| z11b.ibs * IBIS 7.0 Model
| 8Gb DDR4 SDRAM - Die Revision "E"
| This Model is valid for Commercial Temperature Range 0C<=Tc<=95C
| Valid for DDR4-1600/1866/2133/2400/2666/2933/3200 operation
| Models *_3200 are applicable for speed grade 3200 Mbps (-062) and below
| Part Number   VDD/VDDQ   Architecture   Package
| MT40A2G4SA   1.2V/1.2V   2Gb   x 4   78-Ball FBGA
| MT40A1G8SA   1.2V/1.2V   1Gb   x 8   78-Ball FBGA
| MT40A512M16LY   1.2V/1.2V   512Mb x 16   96-Ball FBGA
| MT40A2G4Z11B   1.2V/1.2V   2Gb   x 4   Bare Die
| MT40A1G8Z11B   1.2V/1.2V   1Gb   x 8   Bare Die
| MT40A512M16Z11B   1.2V/1.2V   512Mb x 16   Bare Die
[IBIS Ver]   7.0
[File Name]   z11b.ibs
[Date]   2/27/2023
[File Rev]   2.9.2
[Source]   From silicon level SPICE model at Micron Technology, Inc.
   For support contact your local Micron FAE/Sales contacts
   (more information at https://www.micron.com/support/sales-network)
[Notes]   Revision History:
   Rev 2.9.2: 2/27/2023
   - Updated bare die components and pin mapping tables
   Notes:
   - The DQ_IN_ODT* models contain assumed input thresholds,
   the actual threshold values will depend on the VREFDQ
   level set by training
   - This IBIS file uses the Submodel keyword to model the
   DDR4 On-die Termination(ODT) characteristics.
   - The C_comp value in the DQ I/O model is set to match the
   input state of the DQ I/O as measured from the HSPICE model.
   The C_comp value decreases in the DQ/DQS Input ODT models.
   - L_pin values in the Pin sections are loop inductance and
   include the mutual inductance to appropriate POWER/GND
   return paths.  POWER/GND parasitics are modeled in the
   Package Models.
   - Typ and slow corner V-t curves in the following DQ* models
   are shifted relative to strong corner V-t curve
   to contain all 3 corners within appropriate V-t window
   Models   Typ   Slow   V-t duration
   DQ*_34_3200   -100ps   -250ps   500ps
   DQ*_40_3200   -100ps   -250ps   500ps
   DQ*_48_3200   -100ps   -250ps   500ps
   ALERT_3200   -70ps   -180ps   500ps
   - Due to the shift in typ and slow corner, the V-t curves
   may overlap each other. This does not effect the accuracy
   of the IBIS data.
   - The NF_INPUT Model is for Non-functioning pins in the x4
   package
   - The NF_DQ Model is for Non-functioning DQ pins in the
   x4 package
   See Micron IBIS Model Quality Report and Quality Checklist
   for full IQ details
[Disclaimer]  This software code and all associated documentation, comments
   or other information (collectively "Software") is provided
   "AS IS" without warranty of any kind. MICRON TECHNOLOGY, INC.
   ("MTI") EXPRESSLY DISCLAIMS ALL WARRANTIES EXPRESS OR IMPLIED,
   INCLUDING BUT NOT LIMITED TO, NONINFRINGEMENT OF THIRD PARTY
   RIGHTS, AND ANY IMPLIED WARRANTIES OF MERCHANTABILITY OR
   FITNESS FOR ANY PARTICULAR PURPOSE. MTI DOES NOT WARRANT THAT
   THE SOFTWARE WILL MEET YOUR REQUIREMENTS, OR THAT THE
   OPERATION OF THE SOFTWARE WILL BE UNINTERRUPTED OR ERROR-FREE.
   FURTHERMORE, MTI DOES NOT MAKE ANY REPRESENTATIONS REGARDING
   THE USE OR THE RESULTS OF THE USE OF THE SOFTWARE IN TERMS OF
   ITS CORRECTNESS, ACCURACY, RELIABILITY, OR OTHERWISE. THE
   ENTIRE RISK ARISING OUT OF USE OR PERFORMANCE OF THE SOFTWARE
   REMAINS WITH YOU. IN NO EVENT SHALL MTI, ITS AFFILIATED
   COMPANIES OR THEIR SUPPLIERS BE LIABLE FOR ANY DIRECT,
   INDIRECT, CONSEQUENTIAL, INCIDENTAL, OR SPECIAL DAMAGES
   (INCLUDING, WITHOUT LIMITATION, DAMAGES FOR LOSS OF PROFITS,
   BUSINESS INTERRUPTION, OR LOSS OF INFORMATION) ARISING OUT OF
   YOUR USE OF OR INABILITY TO USE THE SOFTWARE, EVEN IF MTI HAS
   BEEN ADVISED OF THE POSSIBILITY OF SUCH DAMAGES. Because some
   jurisdictions prohibit the exclusion or limitation of
   liability for consequential or incidental damages, the above
   limitation may not apply to you.
[Copyright]   Copyright 2023 Micron Technology, Inc. All rights reserved.
| COMPONENT: MT40A2G4SA (78-Ball FBGA, x4)
[Component]   MT40A2G4SA
[Package Model] z11b_78ball_pkg
[Manufacturer]  Micron Technology,Inc.
[Package]
|   typ   min   max
R_pkg   0.420   0.337   0.508
L_pkg   1.872nH   1.600nH   2.256nH
C_pkg   0.503pF   0.373pF   0.869pF
[Pin]   signal_name   model_name   R_pin   L_pin   C_pin   | TD_pin(ps)   Z_pin
A1   VDD   POWER
A2   VSS   GND
A3   NF   NF_DQ   0.468   1.674nH   0.508pF   | 29.160   57.411
A7   NF   NF_DQ   0.479   1.742nH   0.585pF   | 31.921   54.584
A8   VSS   GND
A9   VSS   GND
B1   VPP   POWER
B2   VDDQ   POWER
B3   DQS_c   DQS   0.483   1.679nH   0.529pF   | 29.803   56.344
B7   DQ1   DQ   0.467   1.632nH   0.584pF   | 30.879   52.837
B8   VDDQ   POWER
B9   ZQ   NC
C1   VDDQ   POWER
C2   DQ0   DQ   0.469   1.610nH   0.574pF   | 30.404   52.960
C3   DQS_t   DQS   0.475   1.798nH   0.476pF   | 29.260   61.450
C7   VDD   POWER
C8   VSS   GND
C9   VDDQ   POWER
D1   VSS   GND
D2   NC   NC
D3   DQ2   DQ   0.471   1.737nH   0.510pF   | 29.758   58.380
D7   DQ3   DQ   0.464   1.678nH   0.578pF   | 31.131   53.899
D8   NC   NC
D9   VSS   GND
E1   VSSL   GND
E2   VDDQ   POWER
E3   NC   NC
E7   NC   NC
E8   VDDQ   POWER
E9   VSS   GND
F1   VDDL   POWER
F2   NC   NC
F3   ODT   INPUT   0.423   2.049nH   0.469pF   | 30.987   66.123
F7   CK_t   CLKIN   0.424   1.731nH   0.474pF   | 28.640   60.452
F8   CK_c   CLKIN   0.419   1.671nH   0.528pF   | 29.696   56.277
F9   VDD   POWER
G1   VSS   GND
G2   NC   NC
G3   CKE   INPUT   0.417   2.095nH   0.424pF   | 29.791   70.324
G7   CS_n   INPUT   0.417   1.902nH   0.442pF   | 29.003   65.579
G8   NC   NC
G9   TEN   INPUT   0.402   2.078nH   0.888pF   | 42.963   48.376
H1   VDD   POWER
H2   WE_n_A14   INPUT   0.406   2.014nH   0.473pF   | 30.864   65.258
H3   ACT_n   INPUT   0.408   1.881nH   0.419pF   | 28.078   66.976
H7   CAS_n_A15   INPUT   0.405   1.965nH   0.393pF   | 27.777   70.734
H8   RAS_n_A16   INPUT   0.412   1.989nH   0.479pF   | 30.861   64.442
H9   VSS   GND
J1   VREFCA   POWER
J2   BG0   INPUT   0.406   1.898nH   0.453pF   | 29.337   64.694
J3   A10   INPUT   0.406   1.830nH   0.393pF   | 26.827   68.213
J7   A12_BC_n   INPUT   0.406   1.941nH   0.378pF   | 27.084   71.672
J8   BG1   INPUT   0.418   2.042nH   0.470pF   | 30.983   65.919
J9   VDD   POWER
K1   VSS   GND
K2   BA0   INPUT   0.409   1.979nH   0.487pF   | 31.052   63.720
K3   A4   INPUT   0.407   1.854nH   0.438pF   | 28.491   65.085
K7   A3   INPUT   0.405   1.944nH   0.427pF   | 28.818   67.441
K8   BA1   INPUT   0.406   2.024nH   0.474pF   | 30.975   65.344
K9   VSS   GND
L1   RESET_n   INPUT   0.352   1.673nH   0.740pF   | 35.197   47.547
L2   A6   INPUT   0.405   1.847nH   0.490pF   | 30.073   61.424
L3   A0   INPUT   0.405   1.689nH   0.426pF   | 26.827   62.951
L7   A1   INPUT   0.409   1.872nH   0.430pF   | 28.361   66.019
L8   A5   INPUT   0.410   1.932nH   0.502pF   | 31.135   62.058
L9   ALERT_n   ALERT   0.348   1.777nH   0.723pF   | 35.847   49.561
M1   VDD   POWER
M2   A8   INPUT   0.409   1.918nH   0.485pF   | 30.505   62.883
M3   A2   INPUT   0.414   1.875nH   0.410pF   | 27.733   67.600
M7   A9   INPUT   0.411   1.946nH   0.399pF   | 27.864   69.857
M8   A7   INPUT   0.410   1.997nH   0.497pF   | 31.507   63.393
M9   VPP   POWER
N1   VSS   GND
N2   A11   INPUT   0.405   1.872nH   0.506pF   | 30.765   60.840
N3   PARITY   INPUT   0.411   1.710nH   0.481pF   | 28.673   59.651
N7   NC   NC
N8   A13   INPUT   0.416   2.062nH   0.486pF   | 31.647   65.172
N9   VDD   POWER
|***********************PIN MAPPING*****************************************
[Pin Mapping]   pulldown_ref   pullup_ref   gnd_clamp_ref   power_clamp_ref ext_ref
A1   NC   VDD
A2   VSS   NC
A3   NC   NC   VSS   VDDQ
A7   NC   NC   VSS   VDDQ
A8   VSS   NC
A9   VSS   NC
B1   NC   VPP
B2   NC   VDDQ
B3   VSS   VDDQ   VSS   VDDQ
B7   VSS   VDDQ   VSS   VDDQ
B8   NC   VDDQ
B9   NC   NC
C1   NC   VDDQ
C2   VSS   VDDQ   VSS   VDDQ
C3   VSS   VDDQ   VSS   VDDQ
C7   NC   VDD
C8   VSS   NC
C9   NC   VDDQ
D1   VSS   NC
D2   NC   NC
D3   VSS   VDDQ   VSS   VDDQ
D7   VSS   VDDQ   VSS   VDDQ
D8   NC   NC
D9   VSS   NC
E1   VSSL   NC
E2   NC   VDDQ
E3   NC   NC
E7   NC   NC
E8   NC   VDDQ
E9   VSS   NC
F1   NC   VDDL
F2   NC   NC
F3   NC   NC   VSS   VDD
F7   NC   NC   VSS   VDD
F8   NC   NC   VSS   VDD
F9   NC   VDD
G1   VSS   NC
G2   NC   NC
G3   NC   NC   VSS   VDD
G7   NC   NC   VSS   VDD
G8   NC   NC
G9   NC   NC   VSS   VDD
H1   NC   VDD
H2   NC   NC   VSS   VDD
H3   NC   NC   VSS   VDD
H7   NC   NC   VSS   VDD
H8   NC   NC   VSS   VDD
H9   VSS   NC
J1   NC   VREFCA
J2   NC   NC   VSS   VDD
J3   NC   NC   VSS   VDD
J7   NC   NC   VSS   VDD
J8   NC   NC   VSS   VDD
J9   NC   VDD
K1   VSS   NC
K2   NC   NC   VSS   VDD
K3   NC   NC   VSS   VDD
K7   NC   NC   VSS   VDD
K8   NC   NC   VSS   VDD
K9   VSS   NC
L1   NC   NC   VSS   VDD
L2   NC   NC   VSS   VDD
L3   NC   NC   VSS   VDD
L7   NC   NC   VSS   VDD
L8   NC   NC   VSS   VDD
L9   VSS   VDDQ   VSS   VDDQ
M1   NC   VDD
M2   NC   NC   VSS   VDD
M3   NC   NC   VSS   VDD
M7   NC   NC   VSS   VDD
M8   NC   NC   VSS   VDD
M9   NC   VPP
N1   VSS   NC
N2   NC   NC   VSS   VDD
N3   NC   NC   VSS   VDD
N7   NC   NC
N8   NC   NC   VSS   VDD
N9   NC   VDD
|**********************DIFF PIN*********************************************
[Diff_pin]   inv_pin   vdiff   tdelay_typ   tdelay_min   tdelay_max
   C3   B3   0.000V   0ns   NA   NA
   F7   F8   0.250V   0ns   NA   NA
| COMPONENT: MT40A1G8SA (78-Ball FBGA, x8)
[Component]   MT40A1G8SA
[Package Model] z11b_78ball_pkg
[Manufacturer]  Micron Technology,Inc.
[Package]
|   typ   min   max
R_pkg   0.420   0.337   0.508
L_pkg   1.872nH   1.600nH   2.256nH
C_pkg   0.503pF   0.373pF   0.869pF
[Pin]   signal_name   model_name   R_pin   L_pin   C_pin   | TD_pin(ps)   Z_pin
A1   VDD   POWER
A2   VSS   GND
A3   TDQS_c   TDQS   0.468   1.674nH   0.508pF   | 29.160   57.411
A7   DM_n_DBI_n_TDQS_t DM_DBI_TDQS   0.479   1.742nH   0.585pF   | 31.921   54.584
A8   VSS   GND
A9   VSS   GND
B1   VPP   POWER
B2   VDDQ   POWER
B3   DQS_c   DQS   0.483   1.679nH   0.529pF   | 29.803   56.344
B7   DQ1   DQ   0.467   1.632nH   0.584pF   | 30.879   52.837
B8   VDDQ   POWER
B9   ZQ   NC
C1   VDDQ   POWER
C2   DQ0   DQ   0.469   1.610nH   0.574pF   | 30.404   52.960
C3   DQS_t   DQS   0.475   1.798nH   0.476pF   | 29.260   61.450
C7   VDD   POWER
C8   VSS   GND
C9   VDDQ   POWER
D1   VSS   GND
D2   DQ4   DQ   0.484   1.646nH   0.583pF   | 30.984   53.119
D3   DQ2   DQ   0.471   1.737nH   0.510pF   | 29.758   58.380
D7   DQ3   DQ   0.464   1.678nH   0.578pF   | 31.131   53.899
D8   DQ5   DQ   0.467   1.577nH   0.552pF   | 29.512   53.455
D9   VSS   GND
E1   VSSL   GND
E2   VDDQ   POWER
E3   DQ6   DQ   0.466   1.677nH   0.573pF   | 30.994   54.107
E7   DQ7   DQ   0.468   1.704nH   0.570pF   | 31.158   54.677
E8   VDDQ   POWER
E9   VSS   GND
F1   VDDL   POWER
F2   NC   NC
F3   ODT   INPUT   0.423   2.049nH   0.469pF   | 30.987   66.123
F7   CK_t   CLKIN   0.424   1.731nH   0.474pF   | 28.640   60.452
F8   CK_c   CLKIN   0.419   1.671nH   0.528pF   | 29.696   56.277
F9   VDD   POWER
G1   VSS   GND
G2   NC   NC
G3   CKE   INPUT   0.417   2.095nH   0.424pF   | 29.791   70.324
G7   CS_n   INPUT   0.417   1.902nH   0.442pF   | 29.003   65.579
G8   NC   NC
G9   TEN   INPUT   0.402   2.078nH   0.888pF   | 42.963   48.376
H1   VDD   POWER
H2   WE_n_A14   INPUT   0.406   2.014nH   0.473pF   | 30.864   65.258
H3   ACT_n   INPUT   0.408   1.881nH   0.419pF   | 28.078   66.976
H7   CAS_n_A15   INPUT   0.405   1.965nH   0.393pF   | 27.777   70.734
H8   RAS_n_A16   INPUT   0.412   1.989nH   0.479pF   | 30.861   64.442
H9   VSS   GND
J1   VREFCA   POWER
J2   BG0   INPUT   0.406   1.898nH   0.453pF   | 29.337   64.694
J3   A10   INPUT   0.406   1.830nH   0.393pF   | 26.827   68.213
J7   A12_BC_n   INPUT   0.406   1.941nH   0.378pF   | 27.084   71.672
J8   BG1   INPUT   0.418   2.042nH   0.470pF   | 30.983   65.919
J9   VDD   POWER
K1   VSS   GND
K2   BA0   INPUT   0.409   1.979nH   0.487pF   | 31.052   63.720
K3   A4   INPUT   0.407   1.854nH   0.438pF   | 28.491   65.085
K7   A3   INPUT   0.405   1.944nH   0.427pF   | 28.818   67.441
K8   BA1   INPUT   0.406   2.024nH   0.474pF   | 30.975   65.344
K9   VSS   GND
L1   RESET_n   INPUT   0.352   1.673nH   0.740pF   | 35.197   47.547
L2   A6   INPUT   0.405   1.847nH   0.490pF   | 30.073   61.424
L3   A0   INPUT   0.405   1.689nH   0.426pF   | 26.827   62.951
L7   A1   INPUT   0.409   1.872nH   0.430pF   | 28.361   66.019
L8   A5   INPUT   0.410   1.932nH   0.502pF   | 31.135   62.058
L9   ALERT_n   ALERT   0.348   1.777nH   0.723pF   | 35.847   49.561
M1   VDD   POWER
M2   A8   INPUT   0.409   1.918nH   0.485pF   | 30.505   62.883
M3   A2   INPUT   0.414   1.875nH   0.410pF   | 27.733   67.600
M7   A9   INPUT   0.411   1.946nH   0.399pF   | 27.864   69.857
M8   A7   INPUT   0.410   1.997nH   0.497pF   | 31.507   63.393
M9   VPP   POWER
N1   VSS   GND
N2   A11   INPUT   0.405   1.872nH   0.506pF   | 30.765   60.840
N3   PARITY   INPUT   0.411   1.710nH   0.481pF   | 28.673   59.651
N7   NC   NC
N8   A13   INPUT   0.416   2.062nH   0.486pF   | 31.647   65.172
N9   VDD   POWER
|***********************PIN MAPPING*****************************************
[Pin Mapping]   pulldown_ref   pullup_ref   gnd_clamp_ref   power_clamp_ref ext_ref
A1   NC   VDD
A2   VSS   NC
A3   VSS   VDDQ   VSS   VDDQ
A7   VSS   VDDQ   VSS   VDDQ
A8   VSS   NC
A9   VSS   NC
B1   NC   VPP
B2   NC   VDDQ
B3   VSS   VDDQ   VSS   VDDQ
B7   VSS   VDDQ   VSS   VDDQ
B8   NC   VDDQ
B9   NC   NC
C1   NC   VDDQ
C2   VSS   VDDQ   VSS   VDDQ
C3   VSS   VDDQ   VSS   VDDQ
C7   NC   VDD
C8   VSS   NC
C9   NC   VDDQ
D1   VSS   NC
D2   VSS   VDDQ   VSS   VDDQ
D3   VSS   VDDQ   VSS   VDDQ
D7   VSS   VDDQ   VSS   VDDQ
D8   VSS   VDDQ   VSS   VDDQ
D9   VSS   NC
E1   VSSL   NC
E2   NC   VDDQ
E3   VSS   VDDQ   VSS   VDDQ
E7   VSS   VDDQ   VSS   VDDQ
E8   NC   VDDQ
E9   VSS   NC
F1   NC   VDDL
F2   NC   NC
F3   NC   NC   VSS   VDD
F7   NC   NC   VSS   VDD
F8   NC   NC   VSS   VDD
F9   NC   VDD
G1   VSS   NC
G2   NC   NC
G3   NC   NC   VSS   VDD
G7   NC   NC   VSS   VDD
G8   NC   NC
G9   NC   NC   VSS   VDD
H1   NC   VDD
H2   NC   NC   VSS   VDD
H3   NC   NC   VSS   VDD
H7   NC   NC   VSS   VDD
H8   NC   NC   VSS   VDD
H9   VSS   NC
J1   NC   VREFCA
J2   NC   NC   VSS   VDD
J3   NC   NC   VSS   VDD
J7   NC   NC   VSS   VDD
J8   NC   NC   VSS   VDD
J9   NC   VDD
K1   VSS   NC
K2   NC   NC   VSS   VDD
K3   NC   NC   VSS   VDD
K7   NC   NC   VSS   VDD
K8   NC   NC   VSS   VDD
K9   VSS   NC
L1   NC   NC   VSS   VDD
L2   NC   NC   VSS   VDD
L3   NC   NC   VSS   VDD
L7   NC   NC   VSS   VDD
L8   NC   NC   VSS   VDD
L9   VSS   VDDQ   VSS   VDDQ
M1   NC   VDD
M2   NC   NC   VSS   VDD
M3   NC   NC   VSS   VDD
M7   NC   NC   VSS   VDD
M8   NC   NC   VSS   VDD
M9   NC   VPP
N1   VSS   NC
N2   NC   NC   VSS   VDD
N3   NC   NC   VSS   VDD
N7   NC   NC
N8   NC   NC   VSS   VDD
N9   NC   VDD
|**********************DIFF PIN*********************************************
[Diff_pin]   inv_pin   vdiff   tdelay_typ   tdelay_min   tdelay_max
   C3   B3   0.000V   0ns   NA   NA
   F7   F8   0.250V   0ns   NA   NA
| COMPONENT: MT40A512M16LY (96-Ball FBGA, x16)
[Component]   MT40A512M16LY
[Package Model] z11b_96ball_pkg
[Manufacturer]  Micron Technology,Inc.
[Package]
|   typ   min   max
R_pkg   0.430   0.345   0.519
L_pkg   1.948nH   1.288nH   2.760nH
C_pkg   0.475pF   0.369pF   0.665pF
[Pin]   signal_name   model_name   R_pin   L_pin   C_pin   | TD_pin(ps)   Z_pin
A1   VDDQ   POWER
A2   VSS   GND
A3   DQ8   DQ   0.435   1.708nH   0.506pF   | 29.401   58.101
A7   UDQS_c   DQS   0.435   1.613nH   0.548pF   | 29.732   54.261
A8   VSS   GND
A9   VDDQ   POWER
B1   VPP   POWER
B2   VSS   GND
B3   VDD   POWER
B7   UDQS_t   DQS   0.431   1.698nH   0.455pF   | 27.789   61.095
B8   DQ9   DQ   0.444   1.692nH   0.500pF   | 29.079   58.204
B9   VDD   POWER
C1   VDDQ   POWER
C2   DQ12   DQ   0.434   1.644nH   0.464pF   | 27.614   59.539
C3   DQ10   DQ   0.432   1.660nH   0.426pF   | 26.574   62.453
C7   DQ11   DQ   0.432   1.597nH   0.468pF   | 27.330   58.445
C8   DQ13   DQ   0.449   1.676nH   0.511pF   | 29.275   57.258
C9   VSS   GND
D1   VDD   POWER
D2   VSS   GND
D3   DQ14   DQ   0.417   1.687nH   0.434pF   | 27.043   62.363
D7   DQ15   DQ   0.434   1.590nH   0.548pF   | 29.510   53.883
D8   VSS   GND
D9   VDDQ   POWER
E1   VSS   GND
E2   UDM_n_UDBI_n   DM_DBI   0.434   1.573nH   0.520pF   | 28.600   54.992
E3   VSS   GND
E7   LDM_n_LDBI_n   DM_DBI   0.384   1.446nH   0.429pF   | 24.892   58.070
E8   VSS   GND
E9   VSS   GND
F1   VSS   GND
F2   VDDQ   POWER
F3   LDQS_c   DQS   0.375   1.350nH   0.426pF   | 23.993   56.264
F7   DQ1   DQ   0.378   1.373nH   0.457pF   | 25.047   54.807
F8   VDDQ   POWER
F9   ZQ   NC
G1   VDDQ   POWER
G2   DQ0   DQ   0.375   1.481nH   0.414pF   | 24.754   59.833
G3   LDQS_t   DQS   0.371   1.308nH   0.409pF   | 23.117   56.575
G7   VDD   POWER
G8   VSS   GND
G9   VDDQ   POWER
H1   VSS   GND
H2   DQ4   DQ   0.379   1.394nH   0.437pF   | 24.675   56.491
H3   DQ2   DQ   0.392   1.395nH   0.417pF   | 24.109   57.850
H7   DQ3   DQ   0.360   1.277nH   0.452pF   | 24.028   53.155
H8   DQ5   DQ   0.377   1.416nH   0.426pF   | 24.571   57.619
H9   VSS   GND
J1   VDDL   POWER
J2   VDDQ   POWER
J3   DQ6   DQ   0.390   1.403nH   0.430pF   | 24.558   57.139
J7   DQ7   DQ   0.378   1.364nH   0.462pF   | 25.109   54.336
J8   VDDQ   POWER
J9   VDD   POWER
K1   VSSL   GND
K2   CKE   INPUT   0.351   1.723nH   0.365pF   | 25.065   68.730
K3   ODT   INPUT   0.360   1.462nH   0.372pF   | 23.327   62.666
K7   CK_t   CLKIN   0.409   1.787nH   0.403pF   | 26.839   66.573
K8   CK_c   CLKIN   0.410   1.665nH   0.506pF   | 29.023   57.378
K9   VSS   GND
L1   VDD   POWER
L2   WE_n_A14   INPUT   0.487   2.355nH   0.479pF   | 33.583   70.132
L3   ACT_n   INPUT   0.451   2.143nH   0.390pF   | 28.914   74.106
L7   CS_n   INPUT   0.362   1.557nH   0.376pF   | 24.205   64.338
L8   RAS_n_A16   INPUT   0.477   2.317nH   0.489pF   | 33.674   68.805
L9   VDD   POWER
M1   VREFCA   POWER
M2   BG0   INPUT   0.479   2.369nH   0.515pF   | 34.945   67.806
M3   A10   INPUT   0.454   2.248nH   0.434pF   | 31.235   71.982
M7   A12_BC_n   INPUT   0.483   2.319nH   0.419pF   | 31.173   74.387
M8   CAS_n_A15   INPUT   0.478   2.348nH   0.480pF   | 33.562   69.951
M9   VSS   GND
N1   VSS   GND
N2   BA0   INPUT   0.479   2.374nH   0.512pF   | 34.857   68.103
N3   A4   INPUT   0.452   2.100nH   0.478pF   | 31.674   66.312
N7   A3   INPUT   0.450   2.185nH   0.410pF   | 29.934   72.983
N8   BA1   INPUT   0.459   2.323nH   0.470pF   | 33.052   70.281
N9   TEN   INPUT   0.492   2.634nH   0.554pF   | 38.186   68.973
P1   RESET_n   INPUT   0.521   2.658nH   0.645pF   | 41.422   64.175
P2   A6   INPUT   0.454   2.238nH   0.535pF   | 34.595   64.690
P3   A0   INPUT   0.464   2.127nH   0.477pF   | 31.865   66.738
P7   A1   INPUT   0.471   2.405nH   0.460pF   | 33.270   72.288
P8   A5   INPUT   0.486   2.545nH   0.504pF   | 35.814   71.053
P9   ALERT_n   ALERT   0.524   2.753nH   0.619pF   | 41.282   66.689
R1   VDD   POWER
R2   A8   INPUT   0.448   2.284nH   0.514pF   | 34.269   66.643
R3   A2   INPUT   0.486   2.382nH   0.508pF   | 34.785   68.473
R7   A9   INPUT   0.465   2.384nH   0.480pF   | 33.818   70.507
R8   A7   INPUT   0.490   2.582nH   0.538pF   | 37.258   69.301
R9   VPP   POWER
T1   VSS   GND
T2   A11   INPUT   0.487   2.401nH   0.569pF   | 36.954   64.970
T3   PARITY   INPUT   0.468   2.023nH   0.549pF   | 33.310   60.727
T7   NC   NC
T8   A13   INPUT   0.484   2.508nH   0.514pF   | 35.911   69.828
T9   VDD   POWER
|***********************PIN MAPPING*****************************************
[Pin Mapping]   pulldown_ref   pullup_ref   gnd_clamp_ref   power_clamp_ref ext_ref
A1   NC   VDDQ
A2   VSS   NC
A3   VSS   VDDQ   VSS   VDDQ
A7   VSS   VDDQ   VSS   VDDQ
A8   VSS   NC
A9   NC   VDDQ
B1   NC   VPP
B2   VSS   NC
B3   NC   VDD
B7   VSS   VDDQ   VSS   VDDQ
B8   VSS   VDDQ   VSS   VDDQ
B9   NC   VDD
C1   NC   VDDQ
C2   VSS   VDDQ   VSS   VDDQ
C3   VSS   VDDQ   VSS   VDDQ
C7   VSS   VDDQ   VSS   VDDQ
C8   VSS   VDDQ   VSS   VDDQ
C9   VSS   NC
D1   NC   VDD
D2   VSS   NC
D3   VSS   VDDQ   VSS   VDDQ
D7   VSS   VDDQ   VSS   VDDQ
D8   VSS   NC
D9   NC   VDDQ
E1   VSS   NC
E2   VSS   VDDQ   VSS   VDDQ
E3   VSS   NC
E7   VSS   VDDQ   VSS   VDDQ
E8   VSS   NC
E9   VSS   NC
F1   VSS   NC
F2   NC   VDDQ
F3   VSS   VDDQ   VSS   VDDQ
F7   VSS   VDDQ   VSS   VDDQ
F8   NC   VDDQ
F9   NC   NC
G1   NC   VDDQ
G2   VSS   VDDQ   VSS   VDDQ
G3   VSS   VDDQ   VSS   VDDQ
G7   NC   VDD
G8   VSS   NC
G9   NC   VDDQ
H1   VSS   NC
H2   VSS   VDDQ   VSS   VDDQ
H3   VSS   VDDQ   VSS   VDDQ
H7   VSS   VDDQ   VSS   VDDQ
H8   VSS   VDDQ   VSS   VDDQ
H9   VSS   NC
J1   NC   VDDL
J2   NC   VDDQ
J3   VSS   VDDQ   VSS   VDDQ
J7   VSS   VDDQ   VSS   VDDQ
J8   NC   VDDQ
J9   NC   VDD
K1   VSSL   NC
K2   NC   NC   VSS   VDD
K3   NC   NC   VSS   VDD
K7   NC   NC   VSS   VDD
K8   NC   NC   VSS   VDD
K9   VSS   NC
L1   NC   VDD
L2   NC   NC   VSS   VDD
L3   NC   NC   VSS   VDD
L7   NC   NC   VSS   VDD
L8   NC   NC   VSS   VDD
L9   NC   VDD
M1   NC   VREFCA
M2   NC   NC   VSS   VDD
M3   NC   NC   VSS   VDD
M7   NC   NC   VSS   VDD
M8   NC   NC   VSS   VDD
M9   VSS   NC
N1   VSS   NC
N2   NC   NC   VSS   VDD
N3   NC   NC   VSS   VDD
N7   NC   NC   VSS   VDD
N8   NC   NC   VSS   VDD
N9   NC   NC   VSS   VDD
P1   NC   NC   VSS   VDD
P2   NC   NC   VSS   VDD
P3   NC   NC   VSS   VDD
P7   NC   NC   VSS   VDD
P8   NC   NC   VSS   VDD
P9   VSS   VDDQ   VSS   VDDQ
R1   NC   VDD
R2   NC   NC   VSS   VDD
R3   NC   NC   VSS   VDD
R7   NC   NC   VSS   VDD
R8   NC   NC   VSS   VDD
R9   NC   VPP
T1   VSS   NC
T2   NC   NC   VSS   VDD
T3   NC   NC   VSS   VDD
T7   NC   NC
T8   NC   NC   VSS   VDD
T9   NC   VDD
|**********************DIFF PIN*********************************************
[Diff_pin]   inv_pin   vdiff   tdelay_typ   tdelay_min   tdelay_max
   B7   A7   0.000V   0ns   NA   NA
   G3   F3   0.000V   0ns   NA   NA
   K7   K8   0.250V   0ns   NA   NA
| COMPONENT: MT40A2G4Z11B (Bare Die, x4)
[Component]   MT40A2G4Z11B
[Manufacturer]  Micron Technology,Inc.
[Package]
|   typ   min   max
R_pkg   0.001   0.001   0.001
L_pkg   0.001nH   0.001nH   0.001nH
C_pkg   0.001pF   0.001pF   0.001pF
[Pin]   signal_name   model_name   R_pin   L_pin   C_pin
1   VDD   POWER
2   VSS   GND
3   VPP   POWER
4   VDDQ   POWER
5   NC   NC
6   VSS   GND
7   NC   NC
8   VDDQ   POWER
9   NC   NC
10   VSS   GND
11   VSS   GND
12   NC   NC
13   VDDQ   POWER
14   NC   NC
15   VSS   GND
16   VDDQ   POWER
17   VDD   POWER
18   VSS   GND
19   NC   NC
20   VDDQ   POWER
21   NC   NC
22   VSS   GND
23   VSS   GND
24   NC   NC
25   VDDQ   POWER
26   NC   NC
27   VSS   GND
28   VSS   GND
29   NC   NC
30   VDDQ   POWER
31   NC   NC
32   VSS   GND
33   VDD   POWER
34   VSS   GND
35   ZQ   NC
36   VDDQ   POWER
37   DQS_c   DQS
38   VSS   GND
39   DQS_t   DQS
40   VDDQ   POWER
41   NC   NC
42   VSS   GND
43   VSS   GND
44   DQ1   DQ
45   VDDQ   POWER
46   DQ3   DQ
47   VSS   GND
48   VDDQ   POWER
49   VDD   POWER
50   VSS   GND
51   DQ0   DQ
52   VDDQ   POWER
53   DQ2   DQ
54   VSS   GND
55   VSS   GND
56   NC   NC
57   VDDQ   POWER
58   NC   NC
59   VSS   GND
60   VSS   GND
61   NC   NC
62   VDDQ   POWER
63   NC   NC
64   VSS   GND
65   VDD   POWER
66   VSS   GND
67   VDD   POWER
68   VDDL   POWER
69   VSSL   GND
70   CK_t   CLKIN
71   CK_c   CLKIN
72   VSS   GND
73   VDD   POWER
74   ODT   INPUT
75   NC   NC
76   CS_n   INPUT
77   NC   NC
78   CKE   INPUT
79   NC   NC
80   RAS_n_A16   INPUT
81   WE_n_A14   INPUT
82   CAS_n_A15   INPUT
83   ACT_n   INPUT
84   BG1   INPUT
85   A10   INPUT
86   A12_BC_n   INPUT
87   BG0   INPUT
88   BA1   INPUT
89   BA0   INPUT
90   A3   INPUT
91   A4   INPUT
92   TEN   INPUT
93   VSS   GND
94   VREFCA   POWER
95   VDD   POWER
96   A5   INPUT
97   A0   INPUT
98   A1   INPUT
99   ALERT_n   ALERT
100   A6   INPUT
101   RESET_n   INPUT
102   A7   INPUT
103   A8   INPUT
104   A9   INPUT
105   A2   INPUT
106   A13   INPUT
107   A11   INPUT
108   PARITY   INPUT
109   VSS   GND
110   VDD   POWER
111   NC   NC
112   NC   NC
113   VPP   POWER
114   NC   NC
115   NC   NC
116   VDD   POWER
117   VSS   GND
|**************************************PIN MAPPING**************************************
[Pin Mapping]   pulldown_ref   pullup_ref   gnd_clamp_ref   power_clamp_ref  ext_ref
1   NC   VDD
2   VSS   NC
3   NC   VPP
4   NC   VDDQ
5   NC   NC
6   VSS   NC
7   NC   NC
8   NC   VDDQ
9   NC   NC
10   VSS   NC
11   VSS   NC
12   NC   NC
13   NC   VDDQ
14   NC   NC
15   VSS   NC
16   NC   VDDQ
17   NC   VDD
18   VSS   NC
19   NC   NC
20   NC   VDDQ
21   NC   NC
22   VSS   NC
23   VSS   NC
24   NC   NC
25   NC   VDDQ
26   NC   NC
27   VSS   NC
28   VSS   NC
29   NC   NC
30   NC   VDDQ
31   NC   NC
32   VSS   NC
33   NC   VDD
34   VSS   NC
35   NC   NC
36   NC   VDDQ
37   VSS   VDDQ   VSS   VDDQ
38   VSS   NC
39   VSS   VDDQ   VSS   VDDQ
40   NC   VDDQ
41   NC   NC
42   VSS   NC
43   VSS   NC
44   VSS   VDDQ   VSS   VDDQ
45   NC   VDDQ
46   VSS   VDDQ   VSS   VDDQ
47   VSS   NC
48   NC   VDDQ
49   NC   VDD
50   VSS   NC
51   VSS   VDDQ   VSS   VDDQ
52   NC   VDDQ
53   VSS   VDDQ   VSS   VDDQ
54   VSS   NC
55   VSS   NC
56   NC   NC
57   NC   VDDQ
58   NC   NC
59   VSS   NC
60   VSS   NC
61   NC   NC
62   NC   VDDQ
63   NC   NC
64   VSS   NC
65   NC   VDD
66   VSS   NC
67   NC   VDD
68   NC   VDDL
69   VSSL   NC
70   NC   NC   VSS   VDD
71   NC   NC   VSS   VDD
72   VSS   NC
73   NC   VDD
74   NC   NC   VSS   VDD
75   NC   NC
76   NC   NC   VSS   VDD
77   NC   NC
78   NC   NC   VSS   VDD
79   NC   NC
80   NC   NC   VSS   VDD
81   NC   NC   VSS   VDD
82   NC   NC   VSS   VDD
83   NC   NC   VSS   VDD
84   NC   NC
85   NC   NC   VSS   VDD
86   NC   NC   VSS   VDD
87   NC   NC   VSS   VDD
88   NC   NC   VSS   VDD
89   NC   NC   VSS   VDD
90   NC   NC   VSS   VDD
91   NC   NC   VSS   VDD
92   NC   NC   VSS   VDD
93   VSS   NC
94   NC   VREFCA
95   NC   VDD
96   NC   NC   VSS   VDD
97   NC   NC   VSS   VDD
98   NC   NC   VSS   VDD
99   VSS   VDDQ   VSS   VDDQ
100   NC   NC   VSS   VDD
101   NC   NC   VSS   VDD
102   NC   NC   VSS   VDD
103   NC   NC   VSS   VDD
104   NC   NC   VSS   VDD
105   NC   NC   VSS   VDD
106   NC   NC   VSS   VDD
107   NC   NC   VSS   VDD
108   NC   NC   VSS   VDD
109   VSS   NC
110   NC   VDD
111   NC   NC
112   NC   NC
113   NC   VPP
114   NC   NC
115   NC   NC
116   NC   VDD
117   VSS   NC
|**********************DIFF PIN*********************************************
[Diff_pin]   inv_pin   vdiff   tdelay_typ   tdelay_min   tdelay_max
   39   37   0.000V   0ns   NA   NA
   70   71   0.250V   0ns   NA   NA
| COMPONENT: MT40A1G8Z11B (Bare Die, x8)
[Component]   MT40A1G8Z11B
[Manufacturer]  Micron Technology,Inc.
[Package]
|   typ   min   max
R_pkg   0.001   0.001   0.001
L_pkg   0.001nH   0.001nH   0.001nH
C_pkg   0.001pF   0.001pF   0.001pF
[Pin]   signal_name   model_name   R_pin   L_pin   C_pin
1   VDD   POWER
2   VSS   GND
3   VPP   POWER
4   VDDQ   POWER
5   NC   NC
6   VSS   GND
7   NC   NC
8   VDDQ   POWER
9   NC   NC
10   VSS   GND
11   VSS   GND
12   NC   NC
13   VDDQ   POWER
14   NC   NC
15   VSS   GND
16   VDDQ   POWER
17   VDD   POWER
18   VSS   GND
19   NC   NC
20   VDDQ   POWER
21   NC   NC
22   VSS   GND
23   VSS   GND
24   NC   NC
25   VDDQ   POWER
26   NC   NC
27   VSS   GND
28   VSS   GND
29   NC   NC
30   VDDQ   POWER
31   NC   NC
32   VSS   GND
33   VDD   POWER
34   VSS   GND
35   ZQ   NC
36   VDDQ   POWER
37   DQS_c   DQS
38   VSS   GND
39   DQS_t   DQS
40   VDDQ   POWER
41   DM_n_DBI_n_TDQS_t  DM_DBI_TDQS
42   VSS   GND
43   VSS   GND
44   DQ1   DQ
45   VDDQ   POWER
46   DQ3   DQ
47   VSS   GND
48   VDDQ   POWER
49   VDD   POWER
50   VSS   GND
51   DQ0   DQ
52   VDDQ   POWER
53   DQ2   DQ
54   VSS   GND
55   VSS   GND
56   DQ5   DQ
57   VDDQ   POWER
58   DQ7   DQ
59   VSS   GND
60   VSS   GND
61   DQ4   DQ
62   VDDQ   POWER
63   DQ6   DQ
64   VSS   GND
65   VDD   POWER
66   VSS   GND
67   VDD   POWER
68   VDDL   POWER
69   VSSL   GND
70   CK_t   CLKIN
71   CK_c   CLKIN
72   VSS   GND
73   VDD   POWER
74   ODT   INPUT
75   NC   NC
76   CS_n   INPUT
77   NC   NC
78   CKE   INPUT
79   NC   NC
80   RAS_n_A16   INPUT
81   WE_n_A14   INPUT
82   CAS_n_A15   INPUT
83   ACT_n   INPUT
84   BG1   INPUT
85   A10   INPUT
86   A12_BC_n   INPUT
87   BG0   INPUT
88   BA1   INPUT
89   BA0   INPUT
90   A3   INPUT
91   A4   INPUT
92   TEN   INPUT
93   VSS   GND
94   VREFCA   POWER
95   VDD   POWER
96   A5   INPUT
97   A0   INPUT
98   A1   INPUT
99   ALERT_n   ALERT
100   A6   INPUT
101   RESET_n   INPUT
102   A7   INPUT
103   A8   INPUT
104   A9   INPUT
105   A2   INPUT
106   A13   INPUT
107   A11   INPUT
108   PARITY   INPUT
109   VSS   GND
110   VDD   POWER
111   NC   NC
112   NC   NC
113   VPP   POWER
114   NC   NC
115   NC   NC
116   VDD   POWER
117   VSS   GND
|**************************************PIN MAPPING**************************************
[Pin Mapping]   pulldown_ref   pullup_ref   gnd_clamp_ref   power_clamp_ref  ext_ref
1   NC   VDD
2   VSS   NC
3   NC   VPP
4   NC   VDDQ
5   NC   NC
6   VSS   NC
7   NC   NC
8   NC   VDDQ
9   NC   NC
10   VSS   NC
11   VSS   NC
12   NC   NC
13   NC   VDDQ
14   NC   NC
15   VSS   NC
16   NC   VDDQ
17   NC   VDD
18   VSS   NC
19   NC   NC
20   NC   VDDQ
21   NC   NC
22   VSS   NC
23   VSS   NC
24   NC   NC
25   NC   VDDQ
26   NC   NC
27   VSS   NC
28   VSS   NC
29   NC   NC
30   NC   VDDQ
31   NC   NC
32   VSS   NC
33   NC   VDD
34   VSS   NC
35   NC   NC
36   NC   VDDQ
37   VSS   VDDQ   VSS   VDDQ
38   VSS   NC
39   VSS   VDDQ   VSS   VDDQ
40   NC   VDDQ
41   VSS   VDDQ   VSS   VDDQ
42   VSS   NC
43   VSS   NC
44   VSS   VDDQ   VSS   VDDQ
45   NC   VDDQ
46   VSS   VDDQ   VSS   VDDQ
47   VSS   NC
48   NC   VDDQ
49   NC   VDD
50   VSS   NC
51   VSS   VDDQ   VSS   VDDQ
52   NC   VDDQ
53   VSS   VDDQ   VSS   VDDQ
54   VSS   NC
55   VSS   NC
56   VSS   VDDQ   VSS   VDDQ
57   NC   VDDQ
58   VSS   VDDQ   VSS   VDDQ
59   VSS   NC
60   VSS   NC
61   VSS   VDDQ   VSS   VDDQ
62   NC   VDDQ
63   VSS   VDDQ   VSS   VDDQ
64   VSS   NC
65   NC   VDD
66   VSS   NC
67   NC   VDD
68   NC   VDDL
69   VSSL   NC
70   NC   NC   VSS   VDD
71   NC   NC   VSS   VDD
72   VSS   NC
73   NC   VDD
74   NC   NC   VSS   VDD
75   NC   NC
76   NC   NC   VSS   VDD
77   NC   NC
78   NC   NC   VSS   VDD
79   NC   NC
80   NC   NC   VSS   VDD
81   NC   NC   VSS   VDD
82   NC   NC   VSS   VDD
83   NC   NC   VSS   VDD
84   NC   NC
85   NC   NC   VSS   VDD
86   NC   NC   VSS   VDD
87   NC   NC   VSS   VDD
88   NC   NC   VSS   VDD
89   NC   NC   VSS   VDD
90   NC   NC   VSS   VDD
91   NC   NC   VSS   VDD
92   NC   NC   VSS   VDD
93   VSS   NC
94   NC   VREFCA
95   NC   VDD
96   NC   NC   VSS   VDD
97   NC   NC   VSS   VDD
98   NC   NC   VSS   VDD
99   VSS   VDDQ   VSS   VDDQ
100   NC   NC   VSS   VDD
101   NC   NC   VSS   VDD
102   NC   NC   VSS   VDD
103   NC   NC   VSS   VDD
104   NC   NC   VSS   VDD
105   NC   NC   VSS   VDD
106   NC   NC   VSS   VDD
107   NC   NC   VSS   VDD
108   NC   NC   VSS   VDD
109   VSS   NC
110   NC   VDD
111   NC   NC
112   NC   NC
113   NC   VPP
114   NC   NC
115   NC   NC
116   NC   VDD
117   VSS   NC
|**********************DIFF PIN*********************************************
[Diff_pin]   inv_pin   vdiff   tdelay_typ   tdelay_min   tdelay_max
   39   37   0.000V   0ns   NA   NA
   70   71   0.250V   0ns   NA   NA
| COMPONENT: MT40A512M16Z11B (Bare Die, x16)
[Component]   MT40A512M16Z11B
[Manufacturer]  Micron Technology,Inc.
[Package]
|   typ   min   max
R_pkg   0.001   0.001   0.001
L_pkg   0.001nH   0.001nH   0.001nH
C_pkg   0.001pF   0.001pF   0.001pF
[Pin]   signal_name   model_name   R_pin   L_pin   C_pin
1   VDD   POWER
2   VSS   GND
3   VPP   POWER
4   VDDQ   POWER
5   UDQS_c   DQS
6   VSS   GND
7   UDQS_t   DQS
8   VDDQ   POWER
9   DQ8   DQ
10   VSS   GND
11   VSS   GND
12   DQ10   DQ
13   VDDQ   POWER
14   DQ12   DQ
15   VSS   GND
16   VDDQ   POWER
17   VDD   POWER
18   VSS   GND
19   DQ9   DQ
20   VDDQ   POWER
21   DQ11   DQ
22   VSS   GND
23   VSS   GND
24   DQ14   DQ
25   VDDQ   POWER
26   UDM_n_UDBI_n   DM_DBI
27   VSS   GND
28   VSS   GND
29   DQ13   DQ
30   VDDQ   POWER
31   DQ15   DQ
32   VSS   GND
33   VDD   POWER
34   VSS   GND
35   ZQ   NC
36   VDDQ   POWER
37   LDQS_c   DQS
38   VSS   GND
39   LDQS_t   DQS
40   VDDQ   POWER
41   LDM_n_LDBI_n   DM_DBI
42   VSS   GND
43   VSS   GND
44   DQ1   DQ
45   VDDQ   POWER
46   DQ3   DQ
47   VSS   GND
48   VDDQ   POWER
49   VDD   POWER
50   VSS   GND
51   DQ0   DQ
52   VDDQ   POWER
53   DQ2   DQ
54   VSS   GND
55   VSS   GND
56   DQ5   DQ
57   VDDQ   POWER
58   DQ7   DQ
59   VSS   GND
60   VSS   GND
61   DQ4   DQ
62   VDDQ   POWER
63   DQ6   DQ
64   VSS   GND
65   VDD   POWER
66   VSS   GND
67   VDD   POWER
68   VDDL   POWER
69   VSSL   GND
70   CK_t   CLKIN
71   CK_c   CLKIN
72   VSS   GND
73   VDD   POWER
74   ODT   INPUT
75   NC   NC
76   CS_n   INPUT
77   NC   NC
78   CKE   INPUT
79   NC   NC
80   RAS_n_A16   INPUT
81   WE_n_A14   INPUT
82   CAS_n_A15   INPUT
83   ACT_n   INPUT
84   NC   NC
85   A10   INPUT
86   A12_BC_n   INPUT
87   BG0   INPUT
88   BA1   INPUT
89   BA0   INPUT
90   A3   INPUT
91   A4   INPUT
92   TEN   INPUT
93   VSS   GND
94   VREFCA   POWER
95   VDD   POWER
96   A5   INPUT
97   A0   INPUT
98   A1   INPUT
99   ALERT_n   ALERT
100   A6   INPUT
101   RESET_n   INPUT
102   A7   INPUT
103   A8   INPUT
104   A9   INPUT
105   A2   INPUT
106   A13   INPUT
107   A11   INPUT
108   PARITY   INPUT
109   VSS   GND
110   VDD   POWER
111   NC   NC
112   NC   NC
113   VPP   POWER
114   NC   NC
115   NC   NC
116   VDD   POWER
117   VSS   GND
|**************************************PIN MAPPING**************************************
[Pin Mapping]   pulldown_ref   pullup_ref   gnd_clamp_ref   power_clamp_ref  ext_ref
1   NC   VDD
2   VSS   NC
3   NC   VPP
4   NC   VDDQ
5   VSS   VDDQ   VSS   VDDQ
6   VSS   NC
7   VSS   VDDQ   VSS   VDDQ
8   NC   VDDQ
9   VSS   VDDQ   VSS   VDDQ
10   VSS   NC
11   VSS   NC
12   VSS   VDDQ   VSS   VDDQ
13   NC   VDDQ
14   VSS   VDDQ   VSS   VDDQ
15   VSS   NC
16   NC   VDDQ
17   NC   VDD
18   VSS   NC
19   VSS   VDDQ   VSS   VDDQ
20   NC   VDDQ
21   VSS   VDDQ   VSS   VDDQ
22   VSS   NC
23   VSS   NC
24   VSS   VDDQ   VSS   VDDQ
25   NC   VDDQ
26   VSS   VDDQ   VSS   VDDQ
27   VSS   NC
28   VSS   NC
29   VSS   VDDQ   VSS   VDDQ
30   NC   VDDQ
31   VSS   VDDQ   VSS   VDDQ
32   VSS   NC
33   NC   VDD
34   VSS   NC
35   NC   NC
36   NC   VDDQ
37   VSS   VDDQ   VSS   VDDQ
38   VSS   NC
39   VSS   VDDQ   VSS   VDDQ
40   NC   VDDQ
41   VSS   VDDQ   VSS   VDDQ
42   VSS   NC
43   VSS   NC
44   VSS   VDDQ   VSS   VDDQ
45   NC   VDDQ
46   VSS   VDDQ   VSS   VDDQ
47   VSS   NC
48   NC   VDDQ
49   NC   VDD
50   VSS   NC
51   VSS   VDDQ   VSS   VDDQ
52   NC   VDDQ
53   VSS   VDDQ   VSS   VDDQ
54   VSS   NC
55   VSS   NC
56   VSS   VDDQ   VSS   VDDQ
57   NC   VDDQ
58   VSS   VDDQ   VSS   VDDQ
59   VSS   NC
60   VSS   NC
61   VSS   VDDQ   VSS   VDDQ
62   NC   VDDQ
63   VSS   VDDQ   VSS   VDDQ
64   VSS   NC
65   NC   VDD
66   VSS   NC
67   NC   VDD
68   NC   VDDL
69   VSSL   NC
70   NC   NC   VSS   VDD
71   NC   NC   VSS   VDD
72   VSS   NC
73   NC   VDD
74   NC   NC   VSS   VDD
75   NC   NC
76   NC   NC   VSS   VDD
77   NC   NC
78   NC   NC   VSS   VDD
79   NC   NC
80   NC   NC   VSS   VDD
81   NC   NC   VSS   VDD
82   NC   NC   VSS   VDD
83   NC   NC   VSS   VDD
84   NC   NC
85   NC   NC   VSS   VDD
86   NC   NC   VSS   VDD
87   NC   NC   VSS   VDD
88   NC   NC   VSS   VDD
89   NC   NC   VSS   VDD
90   NC   NC   VSS   VDD
91   NC   NC   VSS   VDD
92   NC   NC   VSS   VDD
93   VSS   NC
94   NC   VREFCA
95   NC   VDD
96   NC   NC   VSS   VDD
97   NC   NC   VSS   VDD
98   NC   NC   VSS   VDD
99   VSS   VDDQ   VSS   VDDQ
100   NC   NC   VSS   VDD
101   NC   NC   VSS   VDD
102   NC   NC   VSS   VDD
103   NC   NC   VSS   VDD
104   NC   NC   VSS   VDD
105   NC   NC   VSS   VDD
106   NC   NC   VSS   VDD
107   NC   NC   VSS   VDD
108   NC   NC   VSS   VDD
109   VSS   NC
110   NC   VDD
111   NC   NC
112   NC   NC
113   NC   VPP
114   NC   NC
115   NC   NC
116   NC   VDD
117   VSS   NC
|**********************DIFF PIN*********************************************
[Diff_pin]   inv_pin   vdiff   tdelay_typ   tdelay_min   tdelay_max
   7   5   0.000V   0ns   NA   NA
   39   37   0.000V   0ns   NA   NA
   70   71   0.250V   0ns   NA   NA
|   Model Selector
[Model Selector] DQ
DQ_34_3200   34 Ohm Data I/O with no ODT, 1600-3200Mbps
DQ_40_3200   40 Ohm Data I/O with no ODT, 1600-3200Mbps
DQ_48_3200   48 Ohm Data I/O with no ODT, 1600-3200Mbps
DQ_IN_ODTOFF_3200  Data Input with no ODT, 1600-3200Mbps
DQ_IN_ODT34_3200   Data Input with 34ohm ODT, 1600-3200Mbps
DQ_IN_ODT40_3200   Data Input with 40ohm ODT, 1600-3200Mbps
DQ_IN_ODT48_3200   Data Input with 48ohm ODT, 1600-3200Mbps
DQ_IN_ODT60_3200   Data Input with 60ohm ODT, 1600-3200Mbps
DQ_IN_ODT80_3200   Data Input with 80ohm ODT, 1600-3200Mbps
DQ_IN_ODT120_3200  Data Input with 120ohm ODT, 1600-3200Mbps
DQ_IN_ODT240_3200  Data Input with 240ohm ODT, 1600-3200Mbps
[Model Selector] DQS
DQS_34_3200   34 Ohm Data Strobe I/O with no ODT, 1600-3200Mbps
DQS_40_3200   40 Ohm Data Strobe I/O with no ODT, 1600-3200Mbps
DQS_48_3200   48 Ohm Data Strobe I/O with no ODT, 1600-3200Mbps
DQS_IN_ODTOFF_3200 Data Strobe Input with no ODT, 1600-3200Mbps
DQS_IN_ODT34_3200  Data Strobe Input with 34ohm ODT, 1600-3200Mbps
DQS_IN_ODT40_3200  Data Strobe Input with 40ohm ODT, 1600-3200Mbps
DQS_IN_ODT48_3200  Data Strobe Input with 48ohm ODT, 1600-3200Mbps
DQS_IN_ODT60_3200  Data Strobe Input with 60ohm ODT, 1600-3200Mbps
DQS_IN_ODT80_3200  Data Strobe Input with 80ohm ODT, 1600-3200Mbps
DQS_IN_ODT120_3200 Data Strobe Input with 120ohm ODT, 1600-3200Mbps
DQS_IN_ODT240_3200 Data Strobe Input with 240ohm ODT, 1600-3200Mbps
[Model Selector] DM_DBI
DM_ODTOFF_3200   DM Input Model with no ODT, 1600-3200Mbps
DM_ODT34_3200   DM Input Model with 34ohm ODT, 1600-3200Mbps
DM_ODT40_3200   DM Input Model with 40ohm ODT, 1600-3200Mbps
DM_ODT48_3200   DM Input Model with 48ohm ODT, 1600-3200Mbps
DM_ODT60_3200   DM Input Model with 60ohm ODT, 1600-3200Mbps
DM_ODT80_3200   DM Input Model with 80ohm ODT, 1600-3200Mbps
DM_ODT120_3200   DM Input Model with 120ohm ODT, 1600-3200Mbps
DM_ODT240_3200   DM Input Model with 240ohm ODT, 1600-3200Mbps
DQ_34_3200   34 Ohm DBI I/O with no ODT, 1600-3200Mbps
DQ_40_3200   40 Ohm DBI I/O with no ODT, 1600-3200Mbps
DQ_48_3200   48 Ohm DBI I/O with no ODT, 1600-3200Mbps
DQ_IN_ODTOFF_3200  DBI Input with no ODT, 1600-3200Mbps
DQ_IN_ODT34_3200   DBI Input with 34ohm ODT, 1600-3200Mbps
DQ_IN_ODT40_3200   DBI Input with 40ohm ODT, 1600-3200Mbps
DQ_IN_ODT48_3200   DBI Input with 48ohm ODT, 1600-3200Mbps
DQ_IN_ODT60_3200   DBI Input with 60ohm ODT, 1600-3200Mbps
DQ_IN_ODT80_3200   DBI Input with 80ohm ODT, 1600-3200Mbps
DQ_IN_ODT120_3200  DBI Input with 120ohm ODT, 1600-3200Mbps
DQ_IN_ODT240_3200  DBI Input with 240ohm ODT, 1600-3200Mbps
NF_DQ   Non-Functioning DQ Terminator Model
[Model Selector] DM_DBI_TDQS
DM_ODTOFF_3200   DM Input Model with no ODT, 1600-3200Mbps
DM_ODT34_3200   DM Input Model with 34ohm ODT, 1600-3200Mbps
DM_ODT40_3200   DM Input Model with 40ohm ODT, 1600-3200Mbps
DM_ODT48_3200   DM Input Model with 48ohm ODT, 1600-3200Mbps
DM_ODT60_3200   DM Input Model with 60ohm ODT, 1600-3200Mbps
DM_ODT80_3200   DM Input Model with 80ohm ODT, 1600-3200Mbps
DM_ODT120_3200   DM Input Model with 120ohm ODT, 1600-3200Mbps
DM_ODT240_3200   DM Input Model with 240ohm ODT, 1600-3200Mbps
DQ_34_3200   34 Ohm DBI I/O with no ODT, 1600-3200Mbps
DQ_40_3200   40 Ohm DBI I/O with no ODT, 1600-3200Mbps
DQ_48_3200   48 Ohm DBI I/O with no ODT, 1600-3200Mbps
DQ_IN_ODTOFF_3200  DBI Input with no ODT, 1600-3200Mbps
DQ_IN_ODT34_3200   DBI Input with 34ohm ODT, 1600-3200Mbps
DQ_IN_ODT40_3200   DBI Input with 40ohm ODT, 1600-3200Mbps
DQ_IN_ODT48_3200   DBI Input with 48ohm ODT, 1600-3200Mbps
DQ_IN_ODT60_3200   DBI Input with 60ohm ODT, 1600-3200Mbps
DQ_IN_ODT80_3200   DBI Input with 80ohm ODT, 1600-3200Mbps
DQ_IN_ODT120_3200  DBI Input with 120ohm ODT, 1600-3200Mbps
DQ_IN_ODT240_3200  DBI Input with 240ohm ODT, 1600-3200Mbps
TDQS_ODTOFF_3200   TDQS Terminator Model with no ODT, 1600-3200Mbps
TDQS_ODT34_3200   TDQS Terminator Model with 34ohm ODT, 1600-3200Mbps
TDQS_ODT40_3200   TDQS Terminator Model with 40ohm ODT, 1600-3200Mbps
TDQS_ODT48_3200   TDQS Terminator Model with 48ohm ODT, 1600-3200Mbps
TDQS_ODT60_3200   TDQS Terminator Model with 60ohm ODT, 1600-3200Mbps
TDQS_ODT80_3200   TDQS Terminator Model with 80ohm ODT, 1600-3200Mbps
TDQS_ODT120_3200   TDQS Terminator Model with 120ohm ODT, 1600-3200Mbps
TDQS_ODT240_3200   TDQS Terminator Model with 240ohm ODT, 1600-3200Mbps
NF_DQ   Non-Functioning DQ Terminator Model
[Model Selector] TDQS
TDQS_ODTOFF_3200   TDQS Terminator Model with no ODT, 1600-3200Mbps
TDQS_ODT34_3200   TDQS Terminator Model with 34ohm ODT, 1600-3200Mbps
TDQS_ODT40_3200   TDQS Terminator Model with 40ohm ODT, 1600-3200Mbps
TDQS_ODT48_3200   TDQS Terminator Model with 48ohm ODT, 1600-3200Mbps
TDQS_ODT60_3200   TDQS Terminator Model with 60ohm ODT, 1600-3200Mbps
TDQS_ODT80_3200   TDQS Terminator Model with 80ohm ODT, 1600-3200Mbps
TDQS_ODT120_3200   TDQS Terminator Model with 120ohm ODT, 1600-3200Mbps
TDQS_ODT240_3200   TDQS Terminator Model with 240ohm ODT, 1600-3200Mbps
NF_DQ   Non-Functioning DQ Terminator Model
| Sparse Matrix Package Model for z11b_78ball_pkg (x4/x8)
[Define Package Model]  z11b_78ball_pkg
[Manufacturer]   Micron Technology, Inc.
[OEM]   Micron Technology, Inc.
[Description]   z11b package model for 78-ball x4/x8 FBGA
[Number of Pins]   51
[Pin Numbers]
L3  | A0
L7  | A1
M3  | A2
K7  | A3
K3  | A4
L8  | A5
L2  | A6
M8  | A7
M2  | A8
M7  | A9
J3  | A10
N2  | A11
J7  | A12
N8  | A13
H3  | ACT#
L9  | ALERT#
K2  | BA0
K8  | BA1
J2  | BG0
J8  | BG1
H7  | CAS#
G3  | CKE
F8  | CK_C
F7  | CK_T
G7  | CS#
F3  | ODT
N3  | PARITY
H8  | RAS#
L1  | RESET#
H2  | WE#
C2  | DQ0
D3  | DQ2
D2  | DQ4
E3  | DQ6
B3  | DQS-C
C3  | DQS-T
A3  | TDQS-C
A7  | DM#
B7  | DQ1
D7  | DQ3
D8  | DQ5
E7  | DQ7
G9  | TEN
A1  | VDD
B2  | VDDQ_SUBNET_0
B8  | VDDQ_SUBNET_1
B1  | VPP-B1
M9  | VPP-M9
J1  | VREFCA
A9  | VSS
B9  | ZQ
[Model Data]
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[End Model Data]
[End Package Model]
| Sparse Matrix Package Model for z11b_96ball_pkg (x16)
[Define Package Model]  z11b_96ball_pkg
[Manufacturer]   Micron Technology, Inc.
[OEM]   Micron Technology, Inc.
[Description]   z11b package model for 96-ball x16 FBGA
[Number of Pins]   60
[Pin Numbers]
P3  | A0
P7  | A1
R3  | A2
N7  | A3
N3  | A4
P8  | A5
P2  | A6
R8  | A7
R2  | A8
R7  | A9
M3  | A10
T2  | A11
M7  | A12
T8  | A13
L3  | ACT#
P9  | ALERT#
N2  | BA0
N8  | BA1
M2  | BG0
M8  | CAS#
K2  | CKE
K8  | CK_C
K7  | CK_T
L7  | CS#
K3  | ODT
T3  | PARITY
L8  | RAS#
P1  | RESET#
L2  | WE#
G2  | DQ0
F7  | DQ1
H3  | DQ2
H7  | DQ3
H2  | DQ4
H8  | DQ5
J3  | DQ6
J7  | DQ7
A3  | DQ8
B8  | DQ9
C3  | DQ10
C7  | DQ11
C2  | DQ12
C8  | DQ13
D3  | DQ14
D7  | DQ15
E7  | LDM#
F3  | LDQS-C
G3  | LDQS-T
E2  | UDM#
A7  | UDQS-C
B7  | UDQS-T
F9  | ZQ
N9  | TEN
B3  | VDD
J1  | VDDDLL
A9  | VDDQ
B1  | VPP-B1
R9  | VPP-R9
M1  | VREFCA
B2  | VSS
[Model Data]
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[End Model Data]
[End Package Model]
| Models and submodels in the file (49): DQ_34_3200 (I/O), DQ_40_3200 (I/O), DQ_48_3200 (I/O), DQ_IN_ODTOFF_3200 (Input), DQ_IN_ODT34_3200 (Input), DQ_IN_ODT40_3200 (Input), DQ_IN_ODT48_3200 (Input), DQ_IN_ODT60_3200 (Input), DQ_IN_ODT80_3200 (Input), DQ_IN_ODT120_3200 (Input), DQ_IN_ODT240_3200 (Input), DQS_34_3200 (I/O), DQS_40_3200 (I/O), DQS_48_3200 (I/O), DQS_IN_ODTOFF_3200 (Input), DQS_IN_ODT34_3200 (Input), DQS_IN_ODT40_3200 (Input), DQS_IN_ODT48_3200 (Input), DQS_IN_ODT60_3200 (Input), DQS_IN_ODT80_3200 (Input), DQS_IN_ODT120_3200 (Input), DQS_IN_ODT240_3200 (Input), DM_ODTOFF_3200 (Input), DM_ODT34_3200 (Input), DM_ODT40_3200 (Input), DM_ODT48_3200 (Input), DM_ODT60_3200 (Input), DM_ODT80_3200 (Input), DM_ODT120_3200 (Input), DM_ODT240_3200 (Input), TDQS_ODTOFF_3200 (Terminator), TDQS_ODT34_3200 (Terminator), TDQS_ODT40_3200 (Terminator), TDQS_ODT48_3200 (Terminator), TDQS_ODT60_3200 (Terminator), TDQS_ODT80_3200 (Terminator), TDQS_ODT120_3200 (Terminator), TDQS_ODT240_3200 (Terminator), INPUT (Input), CLKIN (Input), ALERT (Open_sink), NF_DQ (Terminator), 34ohm_ODT_3200 (Dynamic_clamp), 40ohm_ODT_3200 (Dynamic_clamp), 48ohm_ODT_3200 (Dynamic_clamp), 60ohm_ODT_3200 (Dynamic_clamp), 80ohm_ODT_3200 (Dynamic_clamp), 120ohm_ODT_3200 (Dynamic_clamp), 240ohm_ODT_3200 (Dynamic_clamp)
